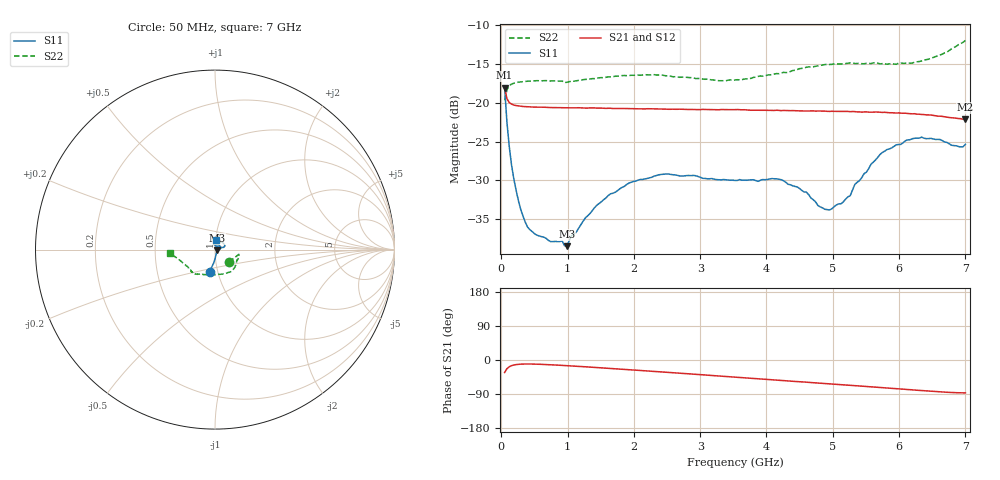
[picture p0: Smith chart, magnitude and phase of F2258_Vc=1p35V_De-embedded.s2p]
! Integrated Device Technology
! Corporate Headquarters
! 6024 Silver Creek Valley Road
! San Jose, CA 95138  USA
! Phone:  1-408-284-8200
! Toll Free:  1-800-223-1366
! Webpage:  http://www.idt.com/
! Timing and RF Division
! 515 Groton Road, Suite 102
! Westford, MA 01886-6024
! Device:  F2258
! Description: Voltage Variable RF Attenuator
! Frequency:  50.0 -  6000.00 MHz
! Package:  3x3 mm Thin QFN Plastic Package: 16 pin
! Ports:  2 RF, 2 DC
!  Pin  1  = NC
!  Pin  2  = NC
!  Pin  3  = RF2  = Port 2
!  Pin  4  = GND
!  Pin  5  = Vdd
!  Pin  6  = NC
!  Pin  7  = VCTRL
!  Pin  8  = NC
!  Pin  9  = GND
!  Pin 10  = RF1  = Port 1
!  Pin 11  = NC
!  Pin 12  = NC
!  Pin 13  = NC
!  Pin 14  = NC
!  Pin 15  = NC
!  Pin 16  = NC
! Vcntrl:  1.350 Volts
! Vdd:  +3.300 Volts
! Current:  1.165 mA
! Data:  The device was measured on a the F2258 evaluation board which has
!  individual transmission lines to the RF pins.  Data was collected
!  using a calibrated network analyzer.  The evaluation board was
!  de-embedded using a TRL calibration technique.
!  The reference plane is the edge of the package pin.
! Misc:  SN 10
!  Action Tracker AT0285
! Date Measured:  2014-12-10
! Date:  2016-01-13  MJV
! Note:
!  Integrated Device Technology supplies this data as a sample of measured
!  data at the package pin for this product.  Your particular data for this
!  product may vary.
!  Data was taken at 25 degrees C.
!  Integrated Device Technology reserves the right to change this data at anytime.
!Freq_(GHz)  S11M_(dB)  S11P_(deg)  S21M_(dB)  S21P_(deg)  S12M_(dB)  S12P_(deg)  S22M_(dB)  S22P_(deg)
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# GHz S dB R 50
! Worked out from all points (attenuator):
!   201 points, 50 MHz to 7 GHz, reference 50 ohm
!   highest |S21| = -18.06 dB at 50 MHz (marker M1); lowest = -22.1 dB at 7 GHz (marker M2)
!   lowest |S11| = -38.4 dB at 988.2 MHz (marker M3), VSWR 1.02, Z = 51.1 - j0.477 ohm
!   |S11| at or under -10 dB: start of sweep to end of sweep
!   |S22| runs from -19.7 to -12.0 dB; largest |S21 - S12| = 0.0009
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0.05  -18.02 -103.7  -18.06 -33.0  -18.08 -33.0  -19.70 -41.6
0.08475  -22.47 -95.8  -19.47 -23.0  -19.49 -23.0  -18.35 -20.3
0.15425  -28.00 -85.9  -20.18 -15.0  -20.18 -15.0  -17.61 -12.9
0.2585  -32.60 -72.8  -20.41 -11.4  -20.41 -11.4  -17.36 -11.4
0.36275  -35.38 -60.2  -20.51 -10.6  -20.49 -10.6  -17.27 -12.6
0.5365  -37.03 -41.9  -20.57 -11.0  -20.54 -11.0  -17.17 -15.5
0.98825  -38.44 -23.0  -20.66 -14.9  -20.60 -14.9  -17.37 -26.4
1.2315  -35.26 -7.3  -20.67 -17.5  -20.61 -17.5  -17.04 -31.7
1.6485  -31.71 3.1  -20.72 -22.4  -20.67 -22.5  -16.67 -40.4
1.9265  -30.33 11.5  -20.76 -25.7  -20.72 -25.7  -16.50 -46.0
2.37825  -29.27 22.8  -20.80 -31.0  -20.78 -31.1  -16.44 -55.7
3.525  -29.99 76.2  -20.89 -45.3  -20.92 -45.2  -17.08 -93.0
4.22  -29.89 100.3  -21.02 -53.9  -21.04 -53.9  -16.20 -117.2
4.7065  -32.48 87.7  -21.05 -59.9  -21.05 -59.9  -15.38 -126.9
4.88025  -33.70 72.2  -21.08 -62.2  -21.06 -62.2  -15.10 -129.0
5.1235  -32.99 44.9  -21.10 -65.1  -21.10 -65.1  -15.03 -131.6
5.2625  -31.96 30.5  -21.15 -66.8  -21.17 -66.8  -14.88 -132.9
5.332  -30.52 25.1  -21.14 -67.8  -21.14 -67.8  -14.97 -133.2
5.57525  -27.93 16.8  -21.22 -70.7  -21.21 -70.7  -14.97 -136.3
5.85325  -25.94 16.0  -21.29 -74.3  -21.27 -74.4  -15.01 -140.6
6.33975  -24.43 24.8  -21.51 -80.8  -21.51 -80.9  -14.63 -152.7
7  -25.35 83.7  -22.14 -86.8  -22.11 -86.9  -12.00 -175.7
